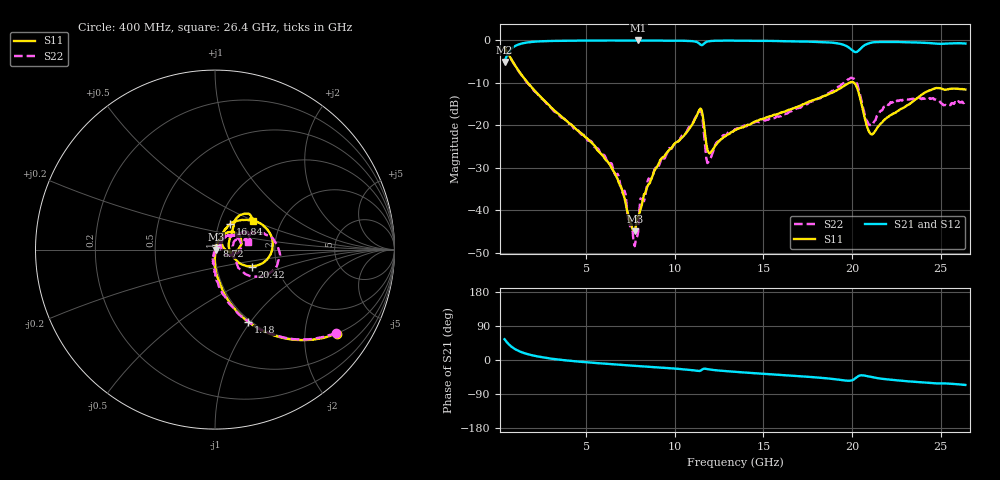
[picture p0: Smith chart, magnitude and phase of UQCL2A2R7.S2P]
! AVX Corporation
! Date:  10/27/06
! Part No:  UQCL2A2R7
! Description:  Ultra Low ESR Microwave capacitors
! Mounting Orientation:  Horizontal
# GHZ S DB R 50
! Freq  |S11|  S11 Ph  |S21|  S21 Ph  |S12|  S12 Ph  |S22|  S22 Ph
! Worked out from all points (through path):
!   401 points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, 400 MHz to 26.4 GHz, reference 50 ohm
!   highest |S21| = -0.01 dB at 7.94 GHz (marker M1); lowest = -5.0 dB at 400 MHz (marker M2)
!   group delay of S21, straight-line fit = 8.73 ps
!   lowest |S11| = -44.9 dB at 7.745 GHz (marker M3), VSWR 1.01, Z = 50.6 + j0.0487 ohm
!   |S11| at or under -10 dB: 1.714 GHz to 19.83 GHz (18.11 GHz wide, 168 % of centre); 20.12 GHz to end of sweep
!   |S22| runs from -48.4 to -1.7 dB; largest |S21 - S12| = 0.016
!   S11 on the Smith chart (normalised r, x): 400 MHz: 0.99, -2.90; 1.18 GHz: 0.97, -0.97; 8.72 GHz: 1.01, +0.05; 16.84 GHz: 1.13, +0.33; 20.42 GHz: 1.48, -0.29; 26.4 GHz: 1.44, +0.49
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0.4  -1.68 -34.7  -5.05 54.7  -5.10 54.7  -1.73 -34.6
1.18  -7.08 -65.3  -0.97 24.1  -1.01 24.1  -7.16 -65.4
2.35  -12.93 -79.7  -0.23 8.7  -0.26 8.8  -13.09 -81.7
4.755  -21.94 -90.1  -0.05 -5.0  -0.06 -4.7  -22.17 -98.2
6.77  -32.52 -85.9  -0.03 -12.3  -0.01 -11.9  -31.39 -107.5
7.55  -43.42 -41.0  -0.03 -14.8  -0.01 -14.4  -43.12 -104.1
7.745  -44.88 4.8  -0.03 -15.4  -0.01 -15.1  -48.40 28.2
7.94  -41.50 29.7  -0.01 -16.1  -0.01 -15.7  -44.99 33.1
8.135  -38.81 58.4  -0.03 -16.9  -0.01 -16.5  -37.37 43.5
8.72  -32.18 71.8  -0.05 -18.5  0.00 -18.1  -32.25 37.5
9.11  -28.87 70.3  -0.05 -19.8  0.00 -19.4  -29.43 47.2
11.385  -16.35 35.8  -0.74 -29.0  -0.71 -29.1  -16.65 21.7
11.905  -26.35 16.1  -0.21 -24.5  -0.18 -24.5  -28.59 22.4
13.4  -21.12 62.0  -0.06 -31.2  -0.02 -31.2  -20.88 51.3
16.845  -15.71 59.5  -0.24 -42.1  -0.18 -42.4  -15.99 32.8
17.755  -14.14 53.9  -0.30 -45.1  -0.24 -45.5  -14.25 28.8
19.9  -9.85 14.6  -1.91 -54.6  -1.86 -55.2  -8.89 -1.8
20.42  -12.93 -24.7  -2.20 -41.3  -2.15 -41.9  -12.24 -37.1
21.07  -22.05 5.1  -0.55 -44.4  -0.50 -45.1  -19.89 3.6
22.11  -17.79 43.3  -0.36 -51.7  -0.32 -52.4  -15.04 31.0
24.645  -11.35 47.6  -0.72 -61.5  -0.69 -62.4  -13.90 17.8
26.4  -11.55 37.1  -0.73 -65.8  -0.71 -66.8  -14.39 13.3
